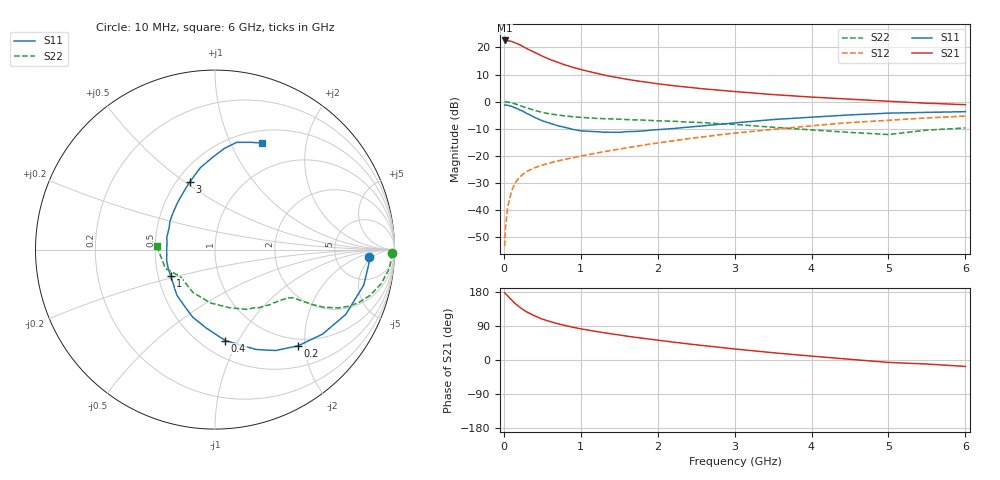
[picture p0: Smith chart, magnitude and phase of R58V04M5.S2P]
! SIEMENS Small Signal Semiconductors
! BFR183
! Si NPN RF Bipolar Junction Transistor in SOT23
! VCE = 8 V  IC = 4.5 mA
! Common Emitter S-Parameters:  May  1996
# GHz  S  MA  R  50
!  f  S11  S21  S12  S22
! GHz  MAG  ANG  MAG  ANG  MAG  ANG  MAG  ANG
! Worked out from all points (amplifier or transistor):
!   36 points, 10 MHz to 6 GHz, reference 50 ohm
!   highest |S21| = 22.6 dB at 10 MHz (marker M1)
!   |S21| within 3 dB of that: start of sweep to 296.8 MHz
!   unconditionally stable (mu >= 1): 1.135 GHz to 2.75 GHz
!   at 250 MHz: K = 0.39, MSG = 23.6 dB, |S12| = -26.9 dB
!   at 1.4 GHz: K = 1.05, MAG = 12.3 dB, |S12| = -18.1 dB
!   at 6 GHz: K = 0.87, MSG = 2.1 dB, |S12| = -5.4 dB
!   S11 on the Smith chart (normalised r, x): 10 MHz: 12, -4; 200 MHz: 0.87, -1.87; 400 MHz: 0.65, -0.88; 1 GHz: 0.58, -0.18; 3 GHz: 0.58, +0.52; 6 GHz: 0.64, +1.32
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0.01  0.8593 -2.6  13.5 177.8  0.0021 83.7  0.9884 -1.2
0.02  0.8608 -5.3  13.31 175.4  0.0044 85.4  0.9837 -2.4
0.05  0.8521 -13.4  13.44 169.0  0.0112 83.3  0.9779 -6.1
0.1  0.8134 -26.3  12.97 158.8  0.022 76.1  0.9449 -11.6
0.15  0.7622 -38.1  12.11 148.6  0.0317 70.7  0.9016 -16.4
0.2  0.7089 -49.1  11.36 140.3  0.0391 65.9  0.8527 -20.3
0.25  0.656 -59.0  10.4 132.8  0.0453 62.0  0.8014 -23.3
0.3  0.601 -67.8  9.502 126.6  0.051 60.4  0.7603 -25.3
0.4  0.5097 -83.6  8.127 116.5  0.0594 57.0  0.6864 -27.9
0.5  0.4389 -96.6  6.911 107.9  0.0664 55.3  0.6279 -29.3
0.6  0.3955 -108.5  6.003 101.6  0.073 54.9  0.59 -30.0
0.7  0.3564 -118.8  5.311 95.8  0.0794 54.8  0.564 -30.6
0.8  0.331 -130.0  4.736 90.9  0.0852 54.8  0.5404 -31.0
1  0.287 -149.7  3.923 82.3  0.0976 56.0  0.5089 -31.8
1.1  0.2808 -158.2  3.614 78.8  0.1041 56.8  0.4976 -32.7
1.6  0.2773 165.6  2.575 62.9  0.139 57.5  0.4631 -37.3
2.2  0.3158 136.2  1.966 47.3  0.1871 56.6  0.4317 -45.6
3  0.4016 110.6  1.532 29.1  0.26 51.3  0.3777 -61.9
3.5  0.4638 100.1  1.344 19.2  0.3055 46.2  0.3339 -76.0
4.5  0.5656 84.8  1.105 1.9  0.4075 35.0  0.2684 -117.3
5.5  0.6296 71.7  0.93 -10.6  0.4969 22.8  0.2956 -159.3
6  0.6485 66.3  0.874 -16.9  0.5385 14.6  0.3242 176.7
